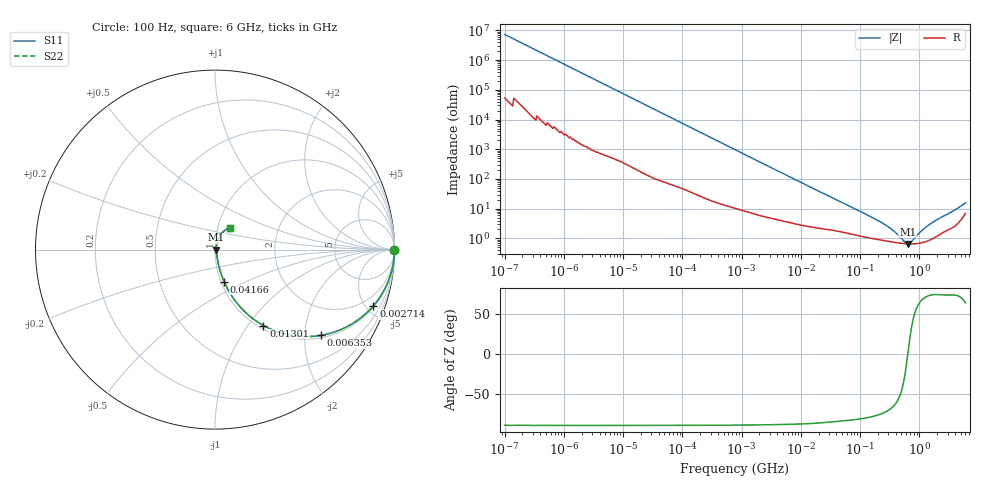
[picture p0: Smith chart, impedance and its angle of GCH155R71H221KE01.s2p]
!Murata Part Number: GCH155R71H221KE01
!These Parameters are Measured in Series Mode Connection
!Data Generated on Jun 19, 2026
!  o--ll--o
!Port1  Port2
!  o------o
!Operation Temp=25[degC], DC Bias Voltage=0[V]
!Freq. Start=100[Hz] Stop=6[GHz] 401[Steps]
# Hz S RI R 50
!Freq.(Hz) S11(Real) S11(Imag) S21(Real) S21(Imag) S12(Real) S12(Imag) S22(Real) S22(Imag)
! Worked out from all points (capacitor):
!   401 points, 100 Hz to 6 GHz, reference 50 ohm
!   read as one part in series: C = 217 pF near 109 Hz
!   lowest |Z| = 656 mohm at 639.6 MHz (marker M1)
!   series resonance near 640.7 MHz, so ESL is about 280 pH
!   S11 on the Smith chart (normalised r, x): 100 Hz: open; 2.714 MHz: 1.10, -5.60; 6.353 MHz: 1.07, -2.41; 13.01 MHz: 1.05, -1.19; 41.66 MHz: 1.04, -0.38; 6 GHz: 1.14, +0.28
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100  1 -1.37e-05  1e-07 1.37e-05  1e-07 1.37e-05  1 -1.37e-05
717  1 -9.72e-05  5e-07 9.72e-05  5e-07 9.72e-05  1 -9.72e-05
2008  1 -0.000272  1.1e-06 0.000272  1.1e-06 0.000272  1 -0.000272
40335  0.9999 -0.00541  5.56e-05 0.00541  5.56e-05 0.00541  0.9999 -0.00541
241822  0.9987 -0.0322  0.00127 0.0322  0.00127 0.0322  0.9987 -0.0322
774597  0.9885 -0.1015  0.0115 0.1015  0.0115 0.1015  0.9885 -0.1015
2713602  0.8825 -0.313  0.1175 0.313  0.1175 0.313  0.8825 -0.313
4060267  0.7741 -0.407  0.2259 0.407  0.2259 0.407  0.7741 -0.407
6353432  0.5904 -0.4778  0.4096 0.4778  0.4096 0.4778  0.5904 -0.4778
1.300572e7  0.27 -0.4232  0.73 0.4232  0.73 0.4232  0.27 -0.4232
1.555665e7  0.2103 -0.3842  0.7897 0.3842  0.7897 0.3842  0.2103 -0.3842
2.434276e7  0.1087 -0.2803  0.8913 0.2803  0.8913 0.2803  0.1087 -0.2803
4.165952e7  0.0506 -0.1779  0.9494 0.1779  0.9494 0.1779  0.0506 -0.1779
1.526266e8  0.0127 -0.0514  0.9873 0.0514  0.9873 0.0514  0.0127 -0.0514
3.124326e8  0.00827 -0.0214  0.9917 0.0214  0.9917 0.0214  0.00827 -0.0214
4.087225e8  0.00733 -0.013  0.9927 0.013  0.9927 0.013  0.00733 -0.013
5.59173e8  0.00665 -0.0039  0.9934 0.0039  0.9934 0.0039  0.00665 -0.0039
6.395615e8  0.00652 -4.92e-05  0.9935 4.92e-05  0.9935 4.92e-05  0.00652 -4.92e-05
7.31507e8  0.0065 0.00385  0.9935 -0.00385  0.9935 -0.00385  0.0065 0.00385
1.094528e9  0.00735 0.0165  0.9927 -0.0165  0.9927 -0.0165  0.00735 0.0165
1.565993e9  0.00992 0.0298  0.9901 -0.0298  0.9901 -0.0298  0.00992 0.0298
6e9  0.0808 0.1206  0.9192 -0.1206  0.9192 -0.1206  0.0808 0.1206
